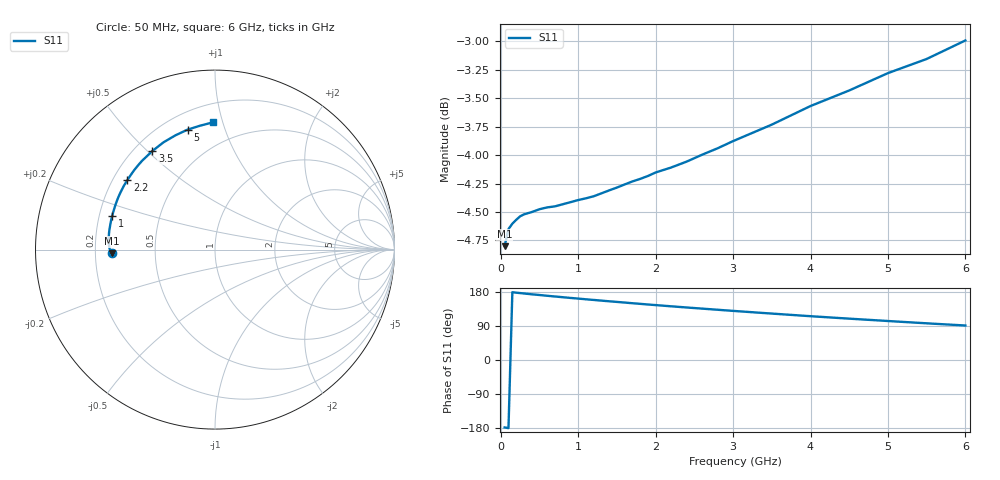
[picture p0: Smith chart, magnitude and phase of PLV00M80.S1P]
! Infineon Technologies  Discrete & RF Semiconductors
! BAR 64-04W /-05W /-06W
! Si PIN Diode in SOT323
! IF = 0.8 mA
! S-Parameters:  October  2008
# GHz  S  MA  R  50
!  f  S11
! GHz  MAG  ANG
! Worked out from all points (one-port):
!   34 points, 50 MHz to 6 GHz, reference 50 ohm
!   lowest |S11| = -4.8 dB at 50 MHz (marker M1), VSWR 3.71, Z = 13.5 - j0.85 ohm
!   |S11| at or under -10 dB: nowhere
!   S11 on the Smith chart (normalised r, x): 50 MHz: 0.27, -0.02; 1 GHz: 0.25, +0.15; 2.2 GHz: 0.26, +0.33; 3.5 GHz: 0.27, +0.52; 5 GHz: 0.30, +0.75; 6 GHz: 0.33, +0.93
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0.05  0.5754 -177.9
0.1  0.5855 -179.8
0.15  0.5887 178.9
0.2  0.591 177.7
0.25  0.5931 176.6
0.4  0.5956 173.4
0.5  0.5974 171.5
0.6  0.5985 169.5
0.8  0.6004 165.7
0.9  0.6016 163.8
1  0.6029 162.1
1.1  0.604 160.2
1.2  0.6052 158.5
1.4  0.6089 154.9
1.6  0.6125 151.6
1.7  0.6144 149.8
1.9  0.6178 146.5
2  0.62 144.9
2.2  0.6231 141.7
2.4  0.6268 138.6
2.6  0.6312 135.6
3  0.64 129.6
3.5  0.6508 122.5
4  0.6631 115.6
4.5  0.6737 109.1
5  0.6856 102.9
5.5  0.6955 96.8
6  0.7086 91.0
